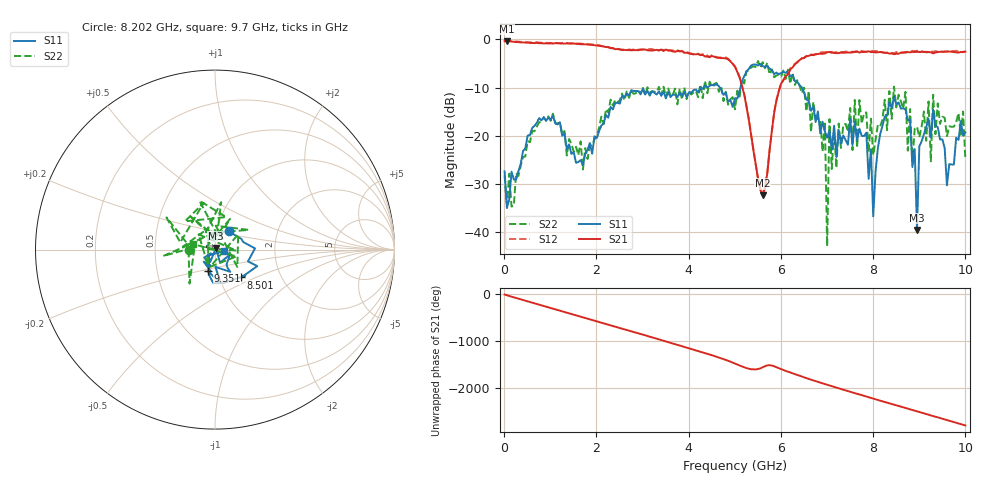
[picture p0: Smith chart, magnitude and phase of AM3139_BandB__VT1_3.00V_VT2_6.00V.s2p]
! Date/Time: Tue, Nov 13, 2018 5:00 PM
! Network Analyzer: Agilent Technologies E8364B Rev: A.07.50.67
! Sweep from 0.010 to 10.000 GHz, 201 Points, Sweep Type: LIN
! Power Supply: 3.001 V, 0.000 A
# Hz S DB R 50
!freq MagS11 AngS11 MagS21 AngS21 MagS12 AngS12 MagS22 AngS22
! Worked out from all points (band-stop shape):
!   201 points, 10 MHz to 10 GHz, reference 50 ohm
!   highest |S21| = -0.31 dB at 59.95 MHz (marker M1); lowest = -32.3 dB at 5.604 GHz (marker M2)
!   |S21| within 3 dB of the highest: start of sweep to 4.319 GHz; 6.631 GHz to end of sweep
!   lowest |S11| = -39.5 dB at 8.951 GHz (marker M3), VSWR 1.02, Z = 50.6 + j0.914 ohm
!   |S11| at or under -10 dB: start of sweep to 4.255 GHz; 4.677 GHz to 5.123 GHz (445.9 MHz wide, 9.1 % of centre); 6.456 GHz to end of sweep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
!   |S22| runs from -42.8 to -4.5 dB; largest |S21 - S12| = 0.032
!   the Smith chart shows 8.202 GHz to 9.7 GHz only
!   S11 on the Smith chart (normalised r, x): 8.202 GHz: 1.14, +0.23; 8.501 GHz: 1.27, -0.41; 9.351 GHz: 0.90, -0.22; 9.7 GHz: 1.10, -0.02
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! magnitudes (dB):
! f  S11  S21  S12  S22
! 10 MHz  -27.3  -0.4  -0.2  -28.1
! 59.95 MHz  -34.9  -0.3  -0.2  -34.8
! 759.2 MHz  -16.3  -0.8  -0.7  -17.2
! 1.708 GHz  -26.0  -1.0  -0.9  -26.9
! 3.357 GHz  -10.8  -2.3  -2.3  -9.8
! 5.005 GHz  -12.2  -5.7  -5.6  -14.5
! 5.604 GHz  -5.5  -32.3  -31.9  -4.7
! 6.703 GHz  -13.9  -3.3  -3.2  -12.9
! 6.953 GHz  -19.0  -2.9  -2.7  -17.0
! 7.003 GHz  -20.4  -2.7  -2.6  -42.8
! 7.053 GHz  -18.9  -2.6  -2.8  -16.5
! 7.852 GHz  -19.3  -2.5  -2.6  -15.1
! 8.002 GHz  -36.6  -2.6  -2.4  -24.0
! 8.202 GHz  -17.9  -2.7  -2.6  -16.6
! 8.352 GHz  -13.0  -3.0  -2.9  -10.7
! 8.501 GHz  -13.4  -3.0  -2.6  -14.1
! 8.801 GHz  -16.7  -2.7  -2.5  -14.4
! 8.951 GHz  -39.5  -2.6  -2.4  -18.1
! 9.001 GHz  -22.1  -2.6  -2.5  -20.3
! 9.351 GHz  -17.9  -2.7  -2.4  -19.6
! 9.7 GHz  -25.9  -2.6  -2.4  -18.1
! 10 GHz  -19.2  -2.5  -2.5  -25.0
